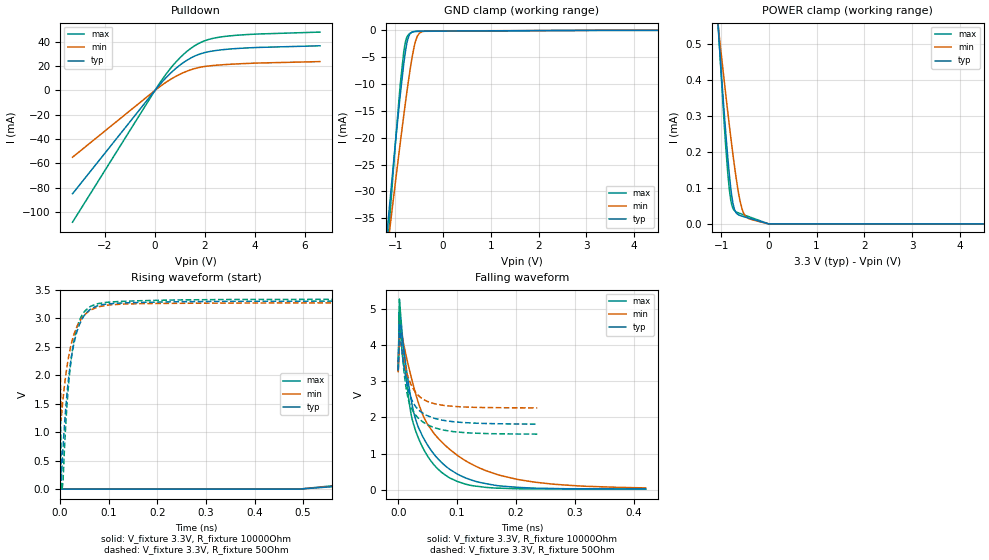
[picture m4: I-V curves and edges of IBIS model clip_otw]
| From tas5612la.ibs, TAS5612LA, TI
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|   clip_otw Model
[Model]   clip_otw
Model_type   Open_drain
Polarity   Inverting
Vmeas = 1.65
Vref = 3.3
Cref = 2pF
Rref = 10000
|   typ   min   max
|   (nom PVT)   (fast PVT)   (slow PVT)
C_comp   8.114e-13   8.085e-13   8.261e-13
|ON state : BUFFER OUTPUT TURNED LOW
|C_comp   8.114e-13   8.085e-13   8.261e-13
|OFF state: BUFFER IN HIGH IMPEDANCE
|C_comp   3.252e-13   2.757e-13   3.645e-13
| Where nom  PVT is Nominal Process, 3.3V, 27C
|   Fast PVT is Strong Process,  3.33V, 0C
|   Slow PVT is Weak Process,   3.27V, 125C
[Voltage Range]   3.3   3.27   3.33
|Ambient Temperature   25   70   0
|Junction Temperature
[Temperature Range]   27   125   0
[Pullup Reference]   3.3   3.27   3.33
[Pulldown Reference]   0   0   0
[Power Clamp Reference]   3.3   3.27   3.33
[GND Clamp Reference]   0   0   0
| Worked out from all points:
|   slope of the pulldown table from 0 to 0.495 V, typ, clamps not added: 42.9 ohm
|   GND clamp passes 1 mA (typ) near -0.72 V on its own axis
|   POWER clamp passes 1 mA (typ) near -1.29 V on its own axis
|   falling waveform, V_fixture 3.3V, R_fixture 10000Ohm: 20-80 % time 58.6ps typ, 96.2ps min, 44.7ps max; typ from 3.3 V to 0.021 V
|   rising waveform, V_fixture 3.3V, R_fixture 10000Ohm: 20-80 % time 4.2ns typ, 5.14ns min, 3.35ns max; typ from 0.018 V to 3.3 V
|   falling waveform, V_fixture 3.3V, R_fixture 50Ohm: 20-80 % time 28.7ps typ, 28.8ps min, 28.1ps max; typ from 3.3 V to 1.81 V
|   rising waveform, V_fixture 3.3V, R_fixture 50Ohm: 20-80 % time 26.6ps typ, 30.7ps min, 22.4ps max; typ from 1.8 V to 3.3 V
[Pulldown]
|   Voltage   I(typ)   I(min)   I(max)
-3.3V     -85.03mA   -54.97mA   -108.4mA
202.2mV   5.008mA    3.215mA    6.411mA
584.8mV   13.4mA     8.582mA    17.2mA
867.9mV   18.66mA    11.93mA    24.02mA
1.15V     23.07mA    14.72mA    29.81mA
1.432V    26.62mA    16.95mA    34.54mA
1.713V    29.29mA    18.6mA     38.22mA
1.995V    31.12mA    19.69mA    40.86mA
2.7V      33.45mA    21.07mA    44.13mA
3.969V    35.2mA     22.38mA    46.22mA
6.6V      36.67mA    23.68mA    47.95mA
[GND Clamp]
|   Voltage   I(typ)   I(min)   I(max)
-3.3V     -216.1mA   -188.1mA   -249.4mA
-1.802V   -97.82mA   -88.04mA   -116.6mA
-1.046V   -25.32mA   -31.7mA    -26.32mA
-914.1mV  -13.35mA   -22.1mA    -11.71mA
-825mV    -6.232mA   -15.85mA   -3.985mA
-785.9mV  -3.709mA   -13.2mA    -2.004mA
-745.8mV  -1.834mA   -10.59mA   -1.033mA
-646.8mV  -316.4uA   -4.856mA   -343uA
-594mV    -189.8uA   -2.549mA   -241.8uA
-542.8mV  -155.5uA   -1.13mA    -202.7uA
-402.6mV  -142.5uA   -180.1uA   -180uA
6.6V      0A         0A         0A
[POWER Clamp]
|   Voltage   I(typ)   I(min)   I(max)
-3.3V     5.287mA    3.463mA    6.313mA
-1.129V   677.4uA    632.8uA    715.7uA
-1.043V   509.2uA    527.2uA    513.6uA
-917.4mV  278.2uA    377.1uA    242.4uA
-825mV    133.2uA    271.4uA    92.66uA
-749.2mV  55.36uA    190.1uA    42.61uA
-697.1mV  33.33uA    138.8uA    34.64uA
-619.3mV  24.38uA    74.48uA    29.88uA
-542.8mV  20.92uA    34.29uA    26.13uA
-474.7mV  18.27uA    19.38uA    22.85uA
-570uV    21.98nA    19.14nA    93.78nA
6.6V      0A         0A         0A
[Ramp]
R_load = 10000
|   typ   min   max
dV/dt_r   1.96937/4.20984e-09   1.94632/5.20716e-09   1.98902/3.32953e-09
dV/dt_f   1.96937/5.86648e-11   1.94632/9.83475e-11   1.98902/4.47644e-11
[Falling Waveform]
V_fixture = 3.3V
V_fixture_min = 3.27V
V_fixture_max = 3.33V
R_fixture = 10000Ohm
|   Time   V(typ)   V(min)   V(max)
0s        3.3V       3.27V      3.33V
2ps       4.92V      4.658V     5.278V
16ps      3.097V     3.524V     2.742V
24ps      2.308V     2.99V      1.926V
34ps      1.735V     2.417V     1.441V
46ps      1.341V     1.922V     1.035V
88ps      558.9mV    1.11V      321.9mV
138ps     204.6mV    601mV      87.93mV
202ps     67.48mV    287.2mV    27.07mV
420ps     21.03mV    50.66mV    15.94mV
[Rising Waveform]
V_fixture = 3.3V
V_fixture_min = 3.27V
V_fixture_max = 3.33V
R_fixture = 10000Ohm
|   Time   V(typ)   V(min)   V(max)
0s        17.72mV    26.13mV    14.97mV
490ps     0V         0V         0V
1.004ns   319.5mV    365.6mV    440.3mV
1.94ns    1.043V     944.4mV    1.319V
3.082ns   1.727V     1.528V     2.068V
4.338ns   2.27V      2.021V     2.597V
5.776ns   2.674V     2.434V     2.948V
8.028ns   3.031V     2.831V     3.204V
10.97ns   3.219V     3.081V     3.308V
18.99ns   3.299V     3.251V     3.332V
[Falling Waveform]
V_fixture = 3.3V
V_fixture_min = 3.27V
V_fixture_max = 3.33V
R_fixture = 50Ohm
|   Time   V(typ)   V(min)   V(max)
0s        3.3V       3.27V      3.33V
2ps       4.605V     4.361V     4.918V
4ps       4.209V     4.102V     4.374V
8ps       3.608V     3.699V     3.547V
14ps      2.998V     3.269V     2.749V
22ps      2.529V     2.903V     2.269V
36ps      2.189V     2.582V     1.952V
60ps      1.985V     2.388V     1.727V
92ps      1.886V     2.311V     1.612V
236ps     1.815V     2.266V     1.54V
[Rising Waveform]
V_fixture = 3.3V
V_fixture_min = 3.27V
V_fixture_max = 3.33V
R_fixture = 50Ohm
|   Time   V(typ)   V(min)   V(max)
0s        1.804V     2.256V     1.534V
2ps       138.6mV    1.204V     0V
6ps       738.8mV    1.588V     152.7mV
14ps      1.666V     2.144V     1.466V
20ps      2.128V     2.435V     2.079V
26ps      2.453V     2.646V     2.48V
40ps      2.892V     2.942V     2.965V
62ps      3.153V     3.137V     3.202V
180ps     3.278V     3.255V     3.308V
778ps     3.299V     3.268V     3.33V
